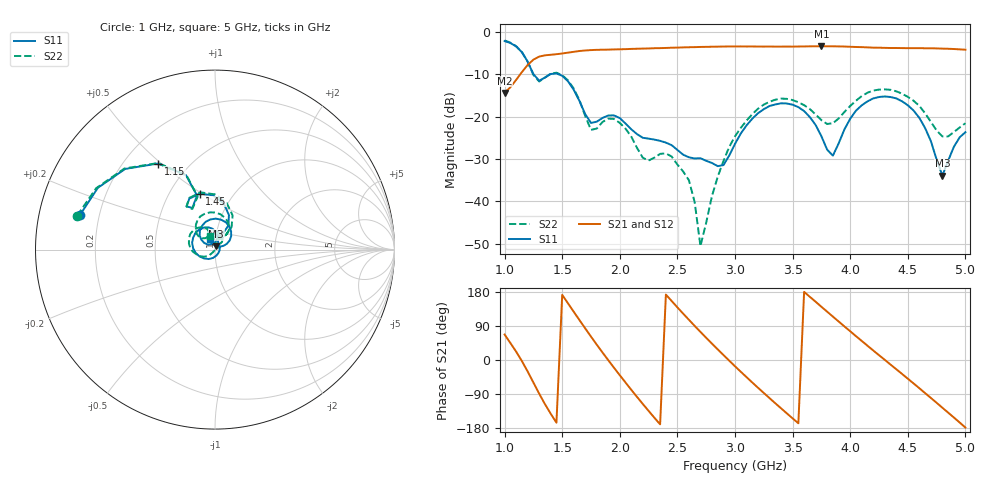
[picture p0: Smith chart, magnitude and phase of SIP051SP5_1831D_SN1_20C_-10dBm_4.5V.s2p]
# GHz  S  dB  R  50
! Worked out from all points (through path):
!   81 points, 1 GHz to 5 GHz, reference 50 ohm
!   highest |S21| = -3.40 dB at 3.75 GHz (marker M1); lowest = -14.4 dB at 1 GHz (marker M2)
!   lowest |S11| = -34.0 dB at 4.8 GHz (marker M3), VSWR 1.04, Z = 50.6 + j1.92 ohm
!   |S11| at or under -10 dB: 1.251 GHz to 1.397 GHz (146.7 MHz wide, 11.1 % of centre); 1.466 GHz to end of sweep
!   |S22| runs from -50.6 to -2.0 dB; largest |S21 - S12| = 0.0041
!   S11 on the Smith chart (normalised r, x): 1 GHz: 0.13, +0.12; 1.15 GHz: 0.34, +0.49; 1.45 GHz: 0.70, +0.49; 5 GHz: 0.94, +0.11
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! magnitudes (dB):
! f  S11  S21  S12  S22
! 1 GHz  -2.2  -14.4  -14.4  -2.0
! 1.15 GHz  -4.8  -9.5  -9.5  -4.8
! 1.3 GHz  -11.6  -5.8  -5.9  -11.7
! 1.45 GHz  -9.8  -5.3  -5.3  -9.7
! 1.7 GHz  -19.5  -4.4  -4.4  -19.9
! 1.75 GHz  -21.5  -4.3  -4.3  -23.1
! 2 GHz  -20.4  -4.1  -4.1  -21.5
! 2.2 GHz  -25.0  -4.0  -4.0  -29.7
! 2.35 GHz  -25.7  -3.9  -3.8  -28.8
! 2.6 GHz  -29.6  -3.6  -3.6  -35.0
! 2.7 GHz  -29.8  -3.6  -3.6  -50.6
! 2.9 GHz  -31.5  -3.5  -3.5  -30.5
! 3 GHz  -26.4  -3.5  -3.4  -24.7
! 3.35 GHz  -17.2  -3.5  -3.5  -16.0
! 3.7 GHz  -22.0  -3.4  -3.4  -19.5
! 3.75 GHz  -24.6  -3.4  -3.4  -20.9
! 3.85 GHz  -29.2  -3.4  -3.4  -21.6
! 4.05 GHz  -18.6  -3.6  -3.6  -16.3
! 4.35 GHz  -15.4  -3.8  -3.8  -13.7
! 4.6 GHz  -20.3  -3.9  -3.9  -17.5
! 4.8 GHz  -34.0  -4.0  -4.0  -24.7
! 5 GHz  -23.7  -4.2  -4.2  -21.6
